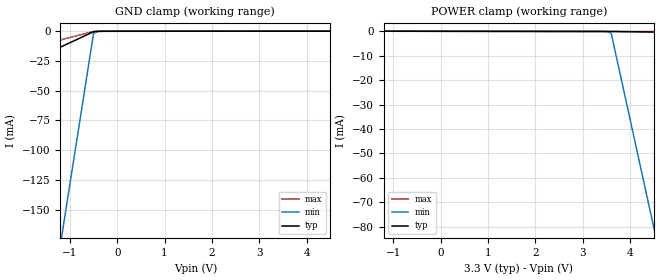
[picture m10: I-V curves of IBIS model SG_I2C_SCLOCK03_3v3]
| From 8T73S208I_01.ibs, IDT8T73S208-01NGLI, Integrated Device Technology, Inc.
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[Model] SG_I2C_SCLOCK03_3v3
Model_type   Input
Polarity   Non-Inverting
Vinl = 0.8V
Vinh = 2.0V
|   typ   min   max
C_comp   2pF   1.5pF   2.5pF
|   typ   min   max
[Voltage range]   3.3V   3.135V   3.465V
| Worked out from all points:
|   GND clamp passes 1 mA (typ) near -0.53 V on its own axis
[GND_clamp]
|Voltage   I (typ)   I (min)   I (max)
-3.3V     -52.32mA   -711.5mA   -28.75mA
-1.2V     -13.41mA   -179.1mA   -7.343mA
-1.1V     -11.55mA   -153.8mA   -6.324mA
-500mV    -433.8uA   -1.689mA   -207.1uA
-400mV    -99.39uA   -184.9uA   -103.3uA
-300mV    -72.6uA    -59.38uA   -98.11uA
6.6V      65.69uA    51.2uA     81.65uA
[Power_clamp]
|Voltage   I (typ)   I (min)   I (max)
-3.3V     65.69uA    48.76uA    85.96uA
3.4V      -67.68uA   -53.33uA   -88.56uA
3.5V      -69.69uA   -104.2uA   -91.17uA
3.6V      -72.6uA    -735.4uA   -93.78uA
4.5V      -313.7uA   -80.22mA   -117.3uA
4.6V      -340.5uA   -89.05mA   -119.9uA
6.6V      -876.2uA   -265.7mA   -172.1uA
